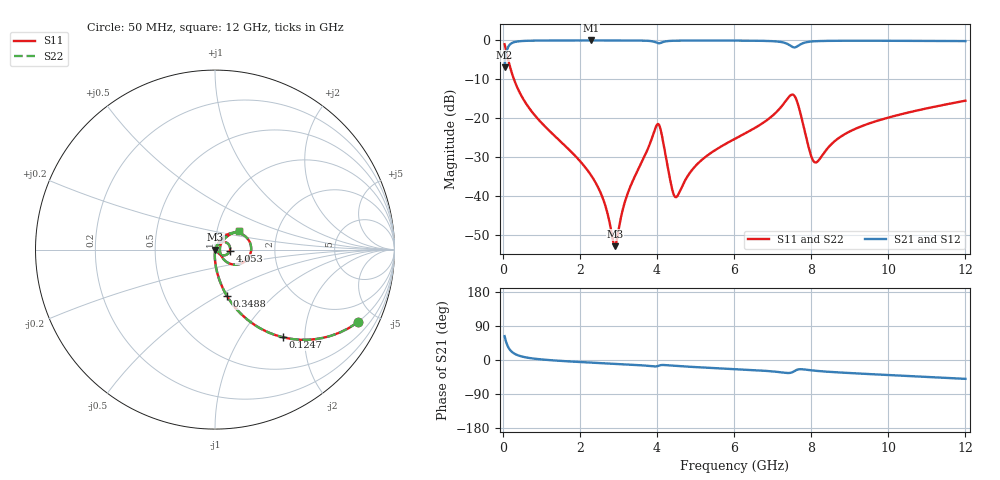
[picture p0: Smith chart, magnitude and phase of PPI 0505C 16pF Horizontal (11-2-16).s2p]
# MHz S MA R 50
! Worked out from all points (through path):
!   1601 points, 50 MHz to 12 GHz, reference 50 ohm
!   highest |S21| = -0.02 dB at 2.283 GHz (marker M1); lowest = -6.9 dB at 50 MHz (marker M2)
!   group delay of S21, straight-line fit = 13.3 ps
!   lowest |S11| = -52.8 dB at 2.911 GHz (marker M3), VSWR 1.00, Z = 50.2 - j0.0425 ohm
!   |S11| at or under -10 dB: 293.2 MHz to end of sweep
!   |S22| runs from -52.8 to -1.0 dB; largest |S21 - S12| = 0
!   S11 on the Smith chart (normalised r, x): 50 MHz: 0.99, -3.92; 124.7 MHz: 0.99, -1.57; 348.8 MHz: 0.99, -0.56; 4.053 GHz: 1.18, -0.02; 12 GHz: 1.27, +0.27
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50  0.8919 -27.1  0.4522 62.9  0.4522 62.9  0.8919 -27.1
124.6875  0.6197 -52.1  0.7845 37.9  0.7845 37.9  0.6197 -52.1
214.3125  0.4163 -66.1  0.9086 23.9  0.9086 23.9  0.4163 -66.1
348.75  0.269 -75.5  0.9624 14.4  0.9624 14.4  0.269 -75.5
841.6875  0.1082 -86.1  0.993 3.3  0.993 3.3  0.1082 -86.1
2044.156  0.02693 -92.0  0.9978 -5.6  0.9978 -5.6  0.02693 -92.0
2283.156  0.01891 -91.4  0.9979 -6.9  0.9979 -6.9  0.01891 -91.4
2611.781  0.009027 -85.7  0.9978 -8.6  0.9978 -8.6  0.009027 -85.7
2910.531  0.002297 -10.6  0.9975 -10.1  0.9975 -10.1  0.002297 -10.6
3261.562  0.01158 62.9  0.9967 -12.0  0.9967 -12.0  0.01158 62.9
4038.312  0.08443 1.7  0.9188 -15.4  0.9188 -15.4  0.08443 1.7
4053.25  0.08281 -4.8  0.9181 -14.9  0.9181 -14.9  0.08281 -4.8
4381.875  0.01319 -30.8  0.987 -15.0  0.987 -15.0  0.01319 -30.8
4493.906  0.009753 7.5  0.9907 -15.8  0.9907 -15.8  0.009753 7.5
5069  0.02657 60.9  0.9947 -19.0  0.9947 -19.0  0.02657 60.9
6025  0.05475 61.0  0.9932 -23.9  0.9932 -23.9  0.05475 61.0
7518.75  0.2017 0.6  0.8236 -31.9  0.8236 -31.9  0.2017 0.6
7660.656  0.1501 -33.6  0.8509 -24.9  0.8509 -24.9  0.1501 -33.6
8019.156  0.03102 -24.2  0.9685 -27.5  0.9685 -27.5  0.03102 -24.2
8146.125  0.0275 8.4  0.9774 -28.7  0.9774 -28.7  0.0275 8.4
10013.31  0.1027 46.9  0.988 -39.7  0.988 -39.7  0.1027 46.9
12000  0.1685 38.2  0.9791 -49.8  0.9791 -49.8  0.1685 38.2
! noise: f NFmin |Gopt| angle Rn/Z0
50  0.0004212  0.8762  1.181  0.0007346
1372  0.004373  0.6988  4.998  0.002834
2701  0.007582  0.6656  9.423  0.00432
4031  0.0582  0.9253  13.96  0.17
5360  0.0154  0.6754  18.34  0.008927
6682  0.02412  0.735  22.71  0.01749
8012  0.05008  0.8394  27.34  0.06236
9341  0.02534  0.6685  31.28  0.01366
1.067e+04  0.0248  0.6277  35.11  0.01141
1.2e+04  0.02638  0.6153  38.87  0.01142
